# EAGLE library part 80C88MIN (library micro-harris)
MICROCONTROLLER/MEMORY DEVICE
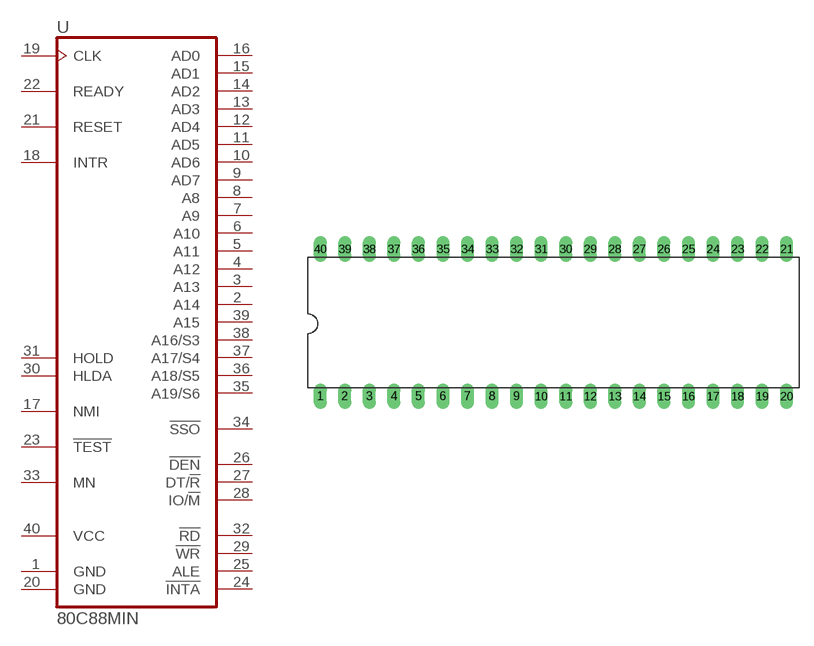
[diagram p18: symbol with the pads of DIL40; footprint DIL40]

Designator prefix U

## 80C88MIN (MF: INTERSIL; MPN: IP80C88-2; OC_FARNELL: unknown; OC_NEWARK: 05B7354)  [DIL40]
1  GND  pwr
2  A14  out
3  A13  out
4  A12  out
5  A11  out
6  A10  out
7  A9  out
8  A8  out
9  AD7
10  AD6
11  AD5
12  AD4
13  AD3
14  AD2
15  AD1
16  AD0
17  NMI  in
18  INTR  in
19  CLK  in
20  GND  pwr
21  RESET  in
22  READY  in
23  !TEST  in
24  !INTA  out
25  ALE  out
26  !DEN  out
27  DT/!R  out
28  IO/!M  out
29  !WR  out
30  HLDA  out
31  HOLD  in
32  !RD  out
33  MN  in
34  !SSO  out
35  A19/S6  out
36  A18/S5  out
37  A17/S4  out
38  A16/S3  out
39  A15  out
40  VCC  pwr

## Footprint DIL40 (pad centres in mm)
Dual In Line Package
drill 0.813 long: 1 -24.13,-7.62; 2 -21.59,-7.62; 3 -19.05,-7.62; 4 -16.51,-7.62; 5 -13.97,-7.62; 6 -11.43,-7.62; 7 -8.89,-7.62; 8 -6.35,-7.62; 9 -3.81,-7.62; 10 -1.27,-7.62; 11 1.27,-7.62; 12 3.81,-7.62; 13 6.35,-7.62; 14 8.89,-7.62; 15 11.43,-7.62; 16 13.97,-7.62; 17 16.51,-7.62; 18 19.05,-7.62; 19 21.59,-7.62; 20 24.13,-7.62; 21 24.13,7.62; 22 21.59,7.62; 23 19.05,7.62; 24 16.51,7.62; 25 13.97,7.62; 26 11.43,7.62; 27 8.89,7.62; 28 6.35,7.62; 29 3.81,7.62; 30 1.27,7.62; 31 -1.27,7.62; 32 -3.81,7.62; 33 -6.35,7.62; 34 -8.89,7.62; 35 -11.43,7.62; 36 -13.97,7.62; 37 -16.51,7.62; 38 -19.05,7.62; 39 -21.59,7.62; 40 -24.13,7.62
